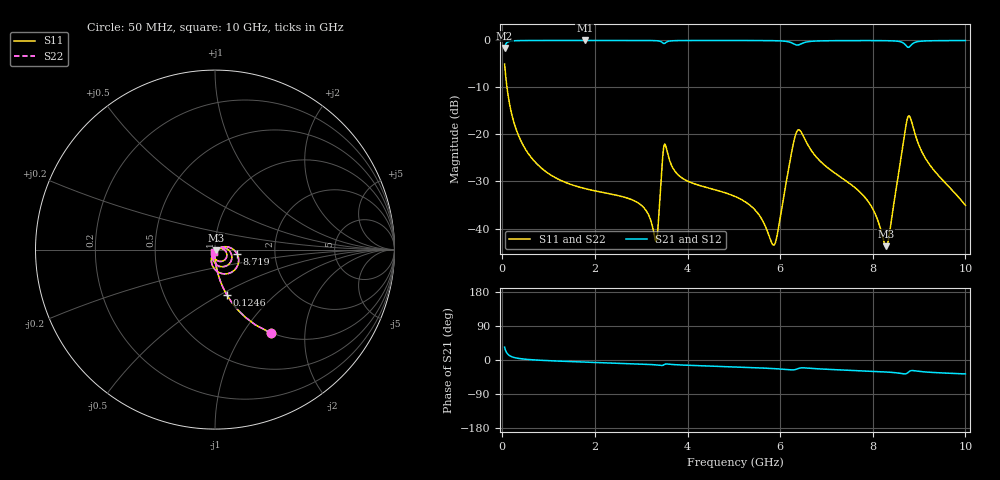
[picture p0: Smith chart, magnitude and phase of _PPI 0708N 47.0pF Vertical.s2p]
! S-Parameter data specifications (vertical orientation):
! Substrate: 40-mil Rogers 3003C, Substrate thickness, H=1.016mm, Dielectric constant, Er=3, Conductor thickness, T_mtl=0.043mm, Loss Tangent, Tand=0.003
! PCB Mounting Pad Footprint: Pad width, PadW=2.54mm , Pad length, PadL=0.51mm , Pad gap, PadG (edge-to-edge)=0.71mm , Reference planes=1.73mm apart
! Created Tue Jan 16 08:53:34 2018
# GHz S MA R 50
! 2 Port Network Data from SP1.SP block
! freq  magS11  angS11  magS21  angS21  magS12  angS12  magS22  angS22
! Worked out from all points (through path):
!   801 points, 50 MHz to 10 GHz, reference 50 ohm
!   highest |S21| = -0.01 dB at 1.779 GHz (marker M1); lowest = -1.6 dB at 50 MHz (marker M2)
!   group delay of S21, straight-line fit = 11.2 ps
!   lowest |S11| = -43.8 dB at 8.284 GHz (marker M3), VSWR 1.01, Z = 50.4 - j0.492 ohm
!   |S11| at or under -10 dB: 101.4 MHz to end of sweep
!   |S22| runs from -43.8 to -5.0 dB; largest |S21 - S12| = 0
!   S11 on the Smith chart (normalised r, x): 50 MHz: 1.00, -1.35; 124.6 MHz: 1.00, -0.54; 8.719 GHz: 1.28, -0.07; 10 GHz: 0.98, -0.03
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0.05  0.5593 -56.2  0.8288 33.8  0.8288 33.8  0.5593 -56.2
0.124625  0.2617 -75.3  0.965 14.7  0.965 14.7  0.2617 -75.3
0.3111875  0.1092 -84.9  0.9938 5.0  0.9938 5.0  0.1092 -84.9
0.622125  0.05709 -88.9  0.9981 0.8  0.9981 0.8  0.05709 -88.9
1.716625  0.02711 -94.3  0.9991 -5.2  0.9991 -5.2  0.02711 -94.3
1.778812  0.02662 -94.5  0.9991 -5.5  0.9991 -5.5  0.02662 -94.5
2.947938  0.01851 -97.4  0.9987 -10.6  0.9987 -10.6  0.01851 -97.4
3.308625  0.007455 -54.7  0.9943 -12.7  0.9943 -12.7  0.007455 -54.7
3.370812  0.01182 1.5  0.9884 -13.4  0.9884 -13.4  0.01182 1.5
3.457875  0.05276 -1.7  0.9483 -14.3  0.9483 -14.3  0.05276 -1.7
3.520062  0.0778 -54.0  0.9417 -10.8  0.9417 -10.8  0.0778 -54.0
3.88075  0.03446 -99.2  0.9968 -13.3  0.9968 -13.3  0.03446 -99.2
5.025  0.02191 -104.5  0.998 -18.4  0.998 -18.4  0.02191 -104.5
5.858313  0.006656 -45.5  0.9936 -22.6  0.9936 -22.6  0.006656 -45.5
6.343375  0.1031 -24.2  0.8966 -24.6  0.8966 -24.6  0.1031 -24.2
6.691625  0.06547 -96.3  0.9798 -22.3  0.9798 -22.3  0.06547 -96.3
7.848312  0.02093 -109.0  0.9958 -28.9  0.9958 -28.9  0.02093 -109.0
8.283625  0.006489 -48.7  0.9935 -31.6  0.9935 -31.6  0.006489 -48.7
8.345812  0.007958 -11.7  0.9922 -32.1  0.9922 -32.1  0.007958 -11.7
8.718937  0.1269 -11.8  0.8828 -36.3  0.8828 -36.3  0.1269 -11.8
8.806  0.1526 -61.1  0.8671 -28.9  0.8671 -28.9  0.1526 -61.1
10  0.01762 -117.5  0.9966 -36.8  0.9966 -36.8  0.01762 -117.5
